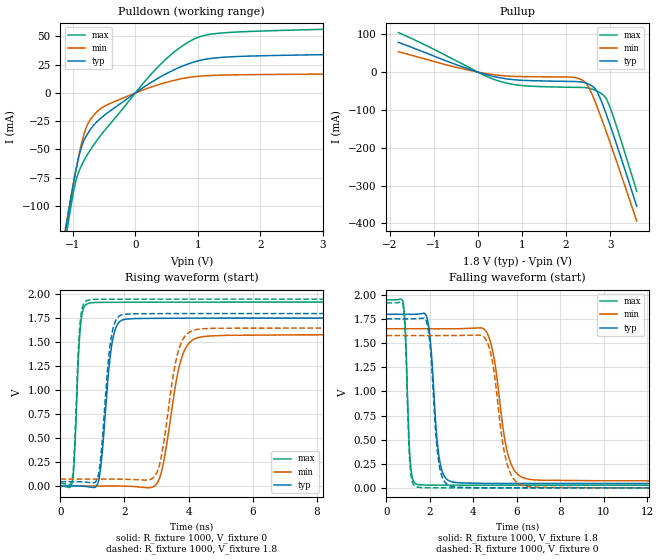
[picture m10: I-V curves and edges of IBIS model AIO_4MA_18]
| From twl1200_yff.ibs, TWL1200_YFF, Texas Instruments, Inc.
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[Model]   AIO_4MA_18
Model_type  Output
Vref =   1.8
Rref =   1M
Cref =   15p
Vmeas =   0.9
| variable   typ   min   max
C_comp   3.81pF   2.79pF   4.80pF
| C_pullup   4.02pF   2.79pF   4.80pF
| C_pulldown   3.61pF   3.11pF   4.17pF
[Temperature Range]   40   100   -40
| Ambient temperature   25   85   -40
[Voltage range]   1.8   1.65   1.95
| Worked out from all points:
|   slope of the pulldown table from 0 to 0.27 V, typ, clamps not added: 27.1 ohm
|   slope of the pullup table from 0 to 0.27 V, typ, clamps not added: 29.8 ohm
|   rising waveform, R_fixture 1000, V_fixture 0: 20-80 % time 268ps typ, 465ps min, 147ps max; typ from 0 V to 1.75 V
|   falling waveform, R_fixture 1000, V_fixture 1.8: 20-80 % time 328ps typ, 586ps min, 174ps max; typ from 1.8 V to 0.045 V
|   rising waveform, R_fixture 1000, V_fixture 1.8: 20-80 % time 258ps typ, 433ps min, 143ps max; typ from 0.045 V to 1.8 V
|   falling waveform, R_fixture 1000, V_fixture 0: 20-80 % time 320ps typ, 565ps min, 165ps max; typ from 1.75 V to 0 V
[Pulldown]
| AIO_4MA_18
|   Voltage   I(typ)   I(min)   I(max)
-1.8V     -370.3mA   -354.5mA   -396.6mA
-1.14V    -129.2mA   -126.6mA   -138.4mA
-1.11V    -118.9mA   -116.8mA   -127.4mA
-1.085V   -110.4mA   -108.8mA   -118.4mA
-965mV    -72.28mA   -71.82mA   -80.71mA
-880mV    -50.99mA   -48.81mA   -66.33mA
-780mV    -37.45mA   -29.7mA    -55.49mA
-650mV    -27.41mA   -18.6mA    -44.64mA
270mV     9.939mA    5.527mA    17.7mA
850mV     25.78mA    13.68mA    45.07mA
1.41V     31.63mA    15.83mA    53.22mA
3.6V      34.37mA    16.86mA    57.13mA
[Pullup]
| AIO_4MA_18
|   Voltage   I(typ)   I(min)   I(max)
-1.8V     78.87mA    54.11mA    104.5mA
-325mV    12.96mA    8.395mA    20.11mA
505mV     -15.01mA   -8.762mA   -24.48mA
1.05V     -21.87mA   -11.9mA    -35.99mA
2.13V     -24.68mA   -13.35mA   -40.12mA
2.395V    -27.3mA    -23.22mA   -40.7mA
2.51V     -31.66mA   -40.02mA   -42.3mA
2.67V     -45.89mA   -82.29mA   -48.47mA
2.77V     -68.71mA   -112.9mA   -54.47mA
2.92V     -114.8mA   -161.3mA   -72.77mA
3.13V     -186.3mA   -231.7mA   -139.3mA
3.6V      -355mA     -394.3mA   -315.4mA
[Ramp]
| AIO_4MA_18
| variable   typ   min   max
dV/dt_r   1.06/2.75E-10   0.96/4.76E-10   1.16/1.53E-10
dV/dt_f   1.06/3.39E-10   0.95/5.91E-10   1.16/1.86E-10
R_load = 1000
[Rising Waveform]
| AIO_4MA_18
R_fixture =   1000
C_fixture =   0
L_fixture =   0
V_fixture =   0
V_fixture_min = 0
V_fixture_max = 0
|   Time   V(typ)   V(min)   V(max)
0s        8.247nV    41.36nV    749.5pV
365ps     704.7uV    -744.6nV   33.77mV
655ps     -240.9uV   -22.95uV   1.754V
1.085ns   -14.22mV   21.53uV    1.915V
1.655ns   1.566V     1.021mV    1.917V
2.325ns   1.747V     -4.921mV   1.918V
3.09ns    1.75V      77.02mV    1.918V
3.93ns    1.751V     1.451V     1.918V
5.17ns    1.752V     1.573V     1.919V
238ns     1.753V     1.579V     1.919V
[Falling Waveform]
| AIO_4MA_18
R_fixture =   1000
C_fixture =   0
L_fixture =   0
V_fixture =   1.8
V_fixture_min = 1.65
V_fixture_max = 1.95
|   Time   V(typ)   V(min)   V(max)
0s        1.8V       1.65V      1.95V
760ps     1.799V     1.65V      1.937V
1.13ns    1.8V       1.65V      195.2mV
1.675ns   1.809V     1.65V      30.01mV
2.495ns   232mV      1.649V     28.13mV
3.405ns   51.76mV    1.65V      27.72mV
4.64ns    46.21mV    1.605V     27.52mV
5.71ns    45.53mV    265mV      27.46mV
7.15ns    45.25mV    78.96mV    27.42mV
238ns     45.1mV     72.71mV    27.4mV
[Rising Waveform]
| AIO_4MA_18
R_fixture =   1000
C_fixture =   0
L_fixture =   0
V_fixture =   1.8
V_fixture_min = 1.65
V_fixture_max = 1.95
|   Time   V(typ)   V(min)   V(max)
0s        45.1mV     72.71mV    27.4mV
390ps     45.84mV    72.71mV    125.2mV
660ps     44.17mV    72.69mV    1.823V
1.09ns    40.65mV    72.77mV    1.948V
1.625ns   1.619V     73mV       1.949V
2.22ns    1.797V     68.83mV    1.949V
3.06ns    1.799V     178.7mV    1.95V
3.825ns   1.799V     1.532V     1.95V
4.83ns    1.8V       1.647V     1.95V
238ns     1.8V       1.65V      1.95V
[Falling Waveform]
| AIO_4MA_18
R_fixture =   1000
C_fixture =   0
L_fixture =   0
V_fixture =   0
V_fixture_min = 0
V_fixture_max = 0
|   Time   V(typ)   V(min)   V(max)
0s        1.753V     1.579V     1.919V
760ps     1.752V     1.579V     1.905V
1.115ns   1.753V     1.579V     162.1mV
1.645ns   1.758V     1.579V     2.161mV
2.48ns    180.5mV    1.579V     615.8uV
3.355ns   5.957mV    1.58V      290.6uV
4.61ns    919.9uV    1.526V     113.5uV
5.625ns   399.2uV    199.3mV    56.45uV
6.99ns    157uV      5.45mV     22.82uV
238ns     30.14nV    52.04nV    17.86nV
